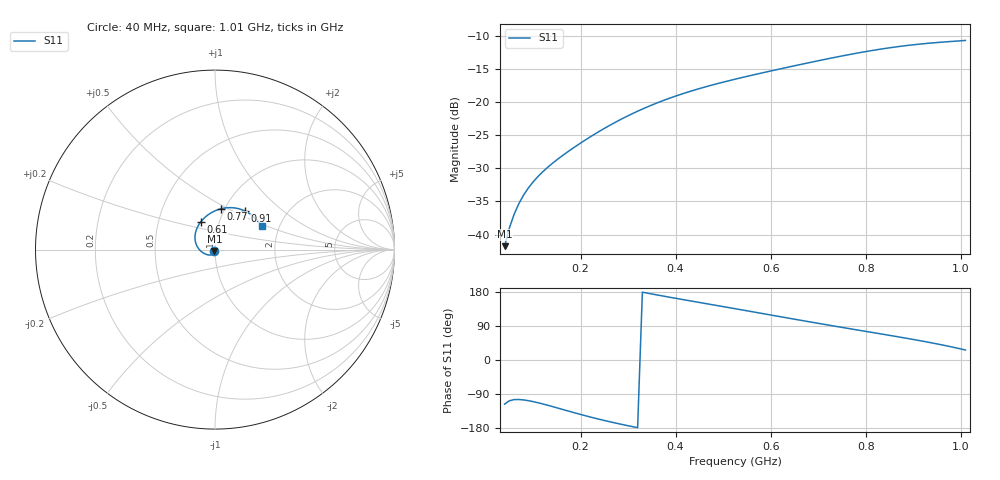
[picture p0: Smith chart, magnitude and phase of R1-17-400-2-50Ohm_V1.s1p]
!version-1
!date-08.2020
!Series
#	GHZ S RI R 50.0
!	FREQ.GHZ	S11RE	S11IM
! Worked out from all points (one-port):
!   98 points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, 40 MHz to 1.01 GHz, reference 50 ohm
!   lowest |S11| = -41.7 dB at 40 MHz (marker M1), VSWR 1.02, Z = 49.6 - j0.728 ohm
!   |S11| at or under -10 dB: start of sweep to end of sweep
!   S11 on the Smith chart (normalised r, x): 40 MHz: 0.99, -0.01; 610 MHz: 0.82, +0.26; 770 MHz: 0.96, +0.46; 910 MHz: 1.25, +0.58; 1.01 GHz: 1.63, +0.46
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0.04  -0.00364 -0.00733
0.05  -0.00337 -0.0107
0.06  -0.00357 -0.0138
0.07  -0.00421 -0.0166
0.08  -0.00526 -0.0192
0.09  -0.00669 -0.0215
0.1  -0.00846 -0.0235
0.12  -0.013 -0.0267
0.14  -0.0185 -0.0289
0.17  -0.0284 -0.0302
0.2  -0.0395 -0.029
0.23  -0.0513 -0.0256
0.26  -0.0632 -0.0199
0.29  -0.0747 -0.012
0.32  -0.0852 -0.0022
0.35  -0.0944 0.00951
0.41  -0.1075 0.0378
0.47  -0.1115 0.0711
0.53  -0.1048 0.1073
0.61  -0.0781 0.156
0.65  -0.0571 0.1785
0.71  -0.0169 0.2074
0.77  0.0323 0.2272
0.83  0.0883 0.2338
0.89  0.1478 0.2229
0.91  0.1678 0.2146
0.96  0.2164 0.1817
1.01  0.2608 0.1293
